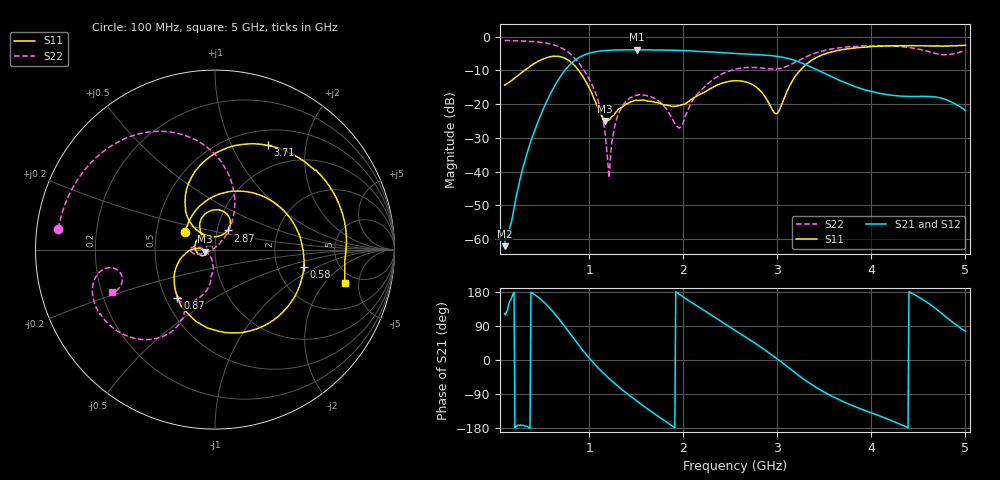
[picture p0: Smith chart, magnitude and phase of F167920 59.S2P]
!  2-Port S-parameters saved by WinCal
! VAR MeasName=S-Parameters (CALIBRATED_DATA) read from VNA (N5242A)
! VAR MeasDate=2016-11-22 9:58:27
! VAR NAME=F167920 59
! VAR FILENAME=F167920 59.S2P
! VAR DATE=2016-11-22 9:58:27
! VAR PHYS_PORTS=1,2
# Hz S DB R 50
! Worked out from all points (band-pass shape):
!   491 points, 100 MHz to 5 GHz, reference 50 ohm
!   highest |S21| = -3.85 dB at 1.51 GHz (marker M1); lowest = -62.2 dB at 100 MHz (marker M2)
!   |S21| within 3 dB of the highest: 853.5 MHz to 3.168 GHz (2.315 GHz wide, 115 % of centre)
!   lowest |S11| = -25.0 dB at 1.17 GHz (marker M3), VSWR 1.12, Z = 44.8 - j1.03 ohm
!   |S11| at or under -10 dB: start of sweep to 310.3 MHz; 887.2 MHz to 3.241 GHz (2.353 GHz wide, 114 % of centre)
!   |S22| runs from -41.8 to -1.1 dB; largest |S21 - S12| = 0.0016
!   S11 on the Smith chart (normalised r, x): 100 MHz: 0.70, +0.14; 580 MHz: 2.82, -0.73; 870 MHz: 0.58, -0.35; 2.87 GHz: 1.12, +0.24; 3.71 GHz: 0.69, +1.39; 5 GHz: 3.95, -3.35
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1e8  -14.36 149.8  -62.17 122.8  -61.47 116.2  -1.10 172.4
3.8e8  -8.61 59.9  -30.89 179.0  -30.93 178.7  -1.38 149.4
5.8e8  -5.95 -11.0  -17.33 136.9  -17.33 137.0  -2.07 127.0
7.3e8  -6.24 -71.1  -10.39 91.7  -10.38 91.8  -3.70 104.1
8.7e8  -9.39 -128.1  -6.54 45.0  -6.54 45.0  -7.15 81.1
9.2e8  -11.20 -146.0  -5.72 29.1  -5.70 29.1  -8.97 73.6
1.08e9  -20.29 176.2  -4.39 -17.0  -4.39 -16.9  -17.70 54.4
1.17e9  -24.97 -168.2  -4.10 -39.3  -4.10 -39.3  -29.02 54.1
1.21e9  -24.77 -157.3  -4.02 -48.6  -4.02 -48.6  -41.85 130.1
1.31e9  -21.54 -156.1  -3.92 -70.1  -3.92 -70.1  -22.85 -161.4
1.51e9  -18.89 166.0  -3.85 -109.1  -3.85 -109.1  -17.41 -177.2
1.74e9  -19.68 132.3  -3.93 -149.7  -3.93 -149.7  -19.10 170.7
1.96e9  -20.44 129.2  -4.03 173.3  -4.04 173.3  -27.04 -138.0
2.15e9  -17.51 128.2  -4.36 142.0  -4.37 142.0  -16.92 -97.7
2.55e9  -13.07 88.7  -4.95 78.6  -4.97 78.5  -9.64 -117.1
2.87e9  -17.85 56.6  -5.45 26.1  -5.46 26.1  -9.40 -128.8
3e9  -22.71 100.9  -5.82 2.6  -5.83 2.6  -9.52 -123.8
3.37e9  -6.89 103.9  -9.11 -65.5  -9.14 -65.5  -5.20 -119.9
3.71e9  -3.73 63.1  -13.51 -110.8  -13.54 -110.6  -3.10 -137.9
4.19e9  -2.70 24.8  -17.27 -157.4  -17.29 -156.9  -2.73 -158.3
4.62e9  -2.73 0.4  -17.73 147.5  -17.73 147.9  -4.49 -170.2
5e9  -2.53 -14.6  -21.85 75.8  -21.85 76.3  -4.14 -157.4
